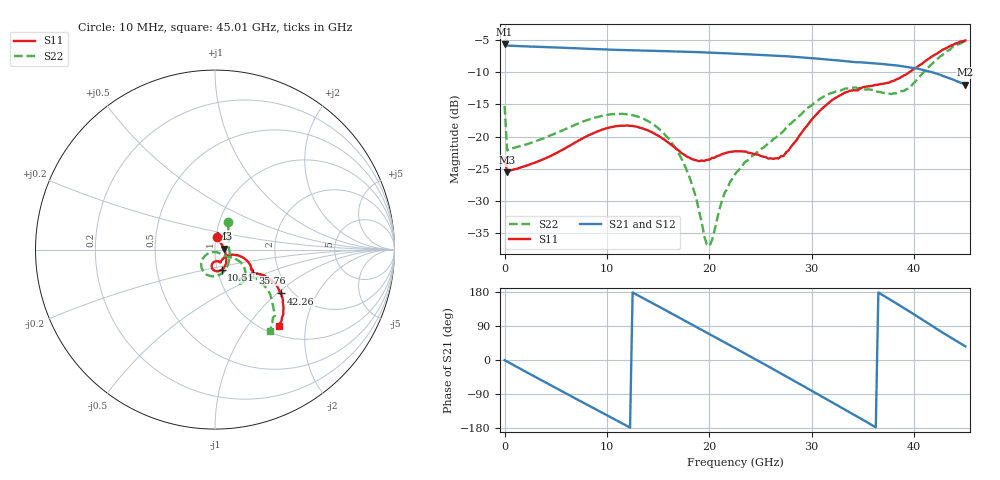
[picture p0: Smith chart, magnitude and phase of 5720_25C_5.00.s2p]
! Device:  ADRF5720
! Description: 0.5dB LSB GaAs MMIC 6-bit Digital Attenuator
! Frequency:  0.000009 -  40 GHz
! Ports:
!	RF1	= Port 1
!	RF2	= Port 2
! Vdd:  3.3 Volt
! Vss:  -3.3 Volt
! Control:  0/3.3 Volt
! State:  5.00 dB attenuation
! Data:  The device was measured using G-S-G Probes on a matrix board.
!  Data was collected using an calibrated 4 port network analyzer.
!  The reference plane for this measurement is at the launchers.
! Note:  Analog Devices supplies this data as a sample of measured data
!  for this product.  Your particular data for this product may vary.
!  Data was taken at 25 degrees C.
!  Analog Devices reserves the right to change this data at anytime.
# GHZ S DB R 45.0
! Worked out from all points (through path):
!   181 points, 10 MHz to 45.01 GHz, reference 45 ohm
!   highest |S21| = -5.73 dB at 10 MHz (marker M1); lowest = -11.9 dB at 45.01 GHz (marker M2)
!   group delay of S21, straight-line fit = 41.8 ps
!   lowest |S11| = -25.5 dB at 260 MHz (marker M3), VSWR 1.11, Z = 50 + j0.509 ohm
!   |S11| at or under -10 dB: start of sweep to 39.57 GHz
!   |S22| runs from -37.0 to -5.3 dB; largest |S21 - S12| = 0.0006
!   S11 on the Smith chart (normalised r, x): 10 MHz: 1.01, +0.14; 10.51 GHz: 1.05, -0.24; 35.76 GHz: 1.47, -0.40; 42.26 GHz: 1.75, -1.06; 45.01 GHz: 1.16, -1.43
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0.01  -23.25 80.5  -5.73 -0.7  -5.74 -0.7  -15.27 65.1
0.26  -25.53 5.5  -5.91 -4.1  -5.92 -4.1  -22.15 2.3
4.26  -23.19 -29.3  -6.16 -62.9  -6.16 -62.9  -19.98 -39.1
7.76  -20.18 -51.2  -6.38 -113.6  -6.38 -113.6  -17.63 -67.7
10.51  -18.51 -71.6  -6.55 -153.1  -6.55 -153.1  -16.54 -91.1
12.76  -18.45 -88.2  -6.66 174.5  -6.66 174.5  -16.79 -111.3
15.26  -20.11 -100.7  -6.75 138.2  -6.75 138.3  -19.04 -133.4
17.76  -23.06 -96.0  -6.87 101.7  -6.87 101.7  -25.09 -149.1
18.76  -23.69 -87.7  -6.92 86.9  -6.92 87.0  -29.81 -145.8
19.51  -23.78 -81.1  -6.97 75.9  -6.97 75.9  -35.47 -125.0
20.01  -23.58 -76.7  -7.00 68.5  -7.00 68.5  -36.98 -87.0
21.51  -22.61 -70.0  -7.10 46.4  -7.10 46.4  -28.67 -37.3
22.76  -22.30 -68.0  -7.19 27.8  -7.19 27.9  -25.37 -32.1
24.76  -22.80 -61.4  -7.34 -1.9  -7.34 -1.9  -22.28 -30.6
26.76  -23.41 -39.2  -7.50 -31.9  -7.50 -31.9  -19.67 -24.9
30.26  -16.92 -14.3  -7.89 -85.2  -7.89 -85.2  -14.80 -29.9
32.76  -13.64 -22.5  -8.24 -123.4  -8.24 -123.4  -12.90 -43.1
35.76  -12.18 -31.4  -8.62 -169.9  -8.63 -169.8  -12.74 -55.9
37.76  -11.48 -30.3  -8.89 158.0  -8.90 158.0  -13.43 -50.2
40.26  -9.28 -28.3  -9.46 115.9  -9.46 115.9  -11.22 -35.2
42.26  -7.13 -33.7  -10.28 81.3  -10.28 81.3  -8.02 -39.2
45.01  -5.12 -50.1  -11.95 36.1  -11.95 36.2  -5.26 -55.8
